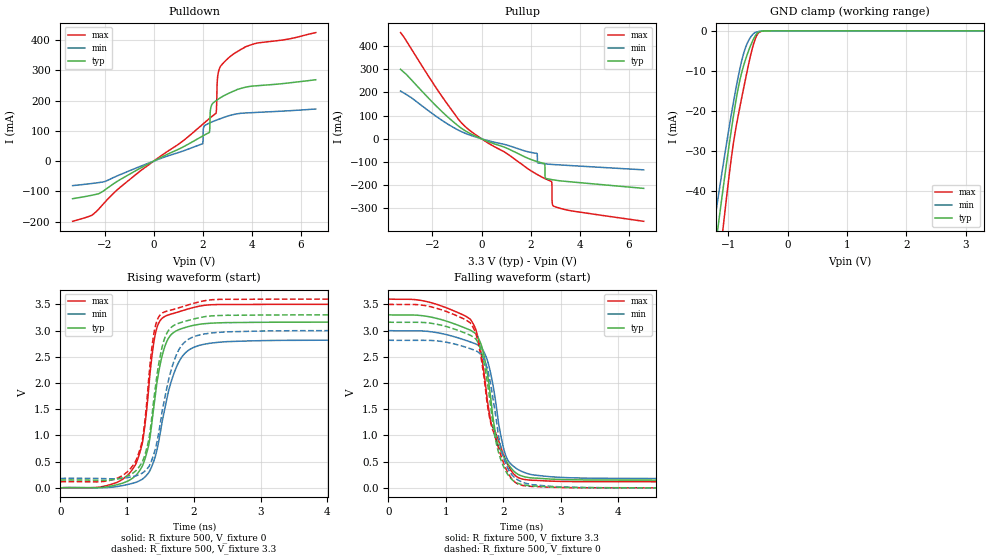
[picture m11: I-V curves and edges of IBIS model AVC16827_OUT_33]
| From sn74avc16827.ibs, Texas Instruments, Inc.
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[Model]   AVC16827_OUT_33
Model_type  3-state
Enable   Active-Low
Vref =   0
Rref =   500
Cref =   30p
Vmeas =   1.5
| variable   typ   min   max
C_comp   4.23pF   3.29pF   5.28pF
| C_pullup   8.79pF   0.04pF   35.28pF
| C_pulldown   16.25pF   1.42pF   50.74pF
| C_tri-state   4.23pF   3.29pF   5.28pF
[Temperature Range]   40   100   -40
| Ambient temperature   25   85   -40
[Voltage range]   3.3   3   3.6
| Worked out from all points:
|   slope of the pulldown table from 0 to 0.495 V, typ, clamps not added: 24.5 ohm
|   slope of the pullup table from 0 to 0.495 V, typ, clamps not added: 23.7 ohm
|   GND clamp passes 1 mA (typ) near -0.53 V on its own axis
|   rising waveform, R_fixture 500, V_fixture 0: 20-80 % time 241ps typ, 309ps min, 207ps max; typ from 0 V to 3.16 V
|   falling waveform, R_fixture 500, V_fixture 3.3: 20-80 % time 293ps typ, 286ps min, 395ps max; typ from 3.3 V to 0.147 V
|   rising waveform, R_fixture 500, V_fixture 3.3: 20-80 % time 223ps typ, 284ps min, 187ps max; typ from 0.147 V to 3.3 V
|   falling waveform, R_fixture 500, V_fixture 0: 20-80 % time 293ps typ, 284ps min, 378ps max; typ from 3.16 V to 0 V
[GND Clamp]
| AVC16827_OUT_33
|   Voltage   I(typ)   I(min)   I(max)
-3.3V     -317.1mA   -273.5mA   -385.8mA
-1.24V    -57.06mA   -48.75mA   -70.66mA
-1.16V    -47.86mA   -40.83mA   -59.48mA
-1.09V    -39.99mA   -34.06mA   -49.94mA
-1.065V   -37.24mA   -31.68mA   -46.61mA
-920mV    -22.15mA   -18.59mA   -28.97mA
-815mV    -13.17mA   -10.31mA   -19.97mA
-695mV    -6.608mA   -3.691mA   -11.11mA
-545mV    -1.293mA   -422.4uA   -2.091mA
-485mV    -308.8uA   -165.9uA   -442.3uA
-370mV    -14.24uA   -20.34uA   -8.566uA
3.3V      1.011nA    10.75nA    48.47pA
[Pulldown]
| AVC16827_OUT_33
|   Voltage   I(typ)   I(min)   I(max)
-3.3V     -124.2mA   -80.91mA   -198.9mA
-2.49V    -112.4mA   -73.57mA   -177.6mA
1.99V     82.86mA    57.31mA    121.5mA
2.04V     85.11mA    112.8mA    125mA
2.265V    94.6mA     125.8mA    140.6mA
2.325V    175.9mA    128.1mA    144.7mA
2.53V     199.3mA    135mA      157.7mA
2.555V    200.8mA    135.7mA    168.3mA
2.59V     202.8mA    136.7mA    264.1mA
2.65V     206.1mA    138.5mA    298.9mA
3.165V    228.4mA    152.5mA    349.4mA
6.6V      269.3mA    172.6mA    425.4mA
[Pullup]
| AVC16827_OUT_33
|   Voltage   I(typ)   I(min)   I(max)
-3.3V     300mA      206.1mA    458.6mA
-735mV    39.21mA    26.92mA    59.95mA
2.255V    -98.1mA    -63.13mA   -153.5mA
2.28V     -98.9mA    -103mA     -155mA
2.565V    -106.8mA   -107.8mA   -170.9mA
2.595V    -168.1mA   -108.1mA   -172.4mA
2.85V     -176mA     -110.5mA   -184.7mA
2.865V    -176.3mA   -110.6mA   -197.1mA
2.87V     -176.4mA   -110.7mA   -265.4mA
2.875V    -176.5mA   -110.7mA   -275.7mA
2.925V    -177.3mA   -111.1mA   -290.3mA
6.6V      -213.9mA   -134mA     -356.1mA
[Ramp]
| AVC16827_OUT_33
| variable   typ   min   max
dV/dt_r   1.90/2.48E-10   1.69/3.13E-10   2.10/2.13E-10
dV/dt_f   1.89/3.01E-10   1.69/2.87E-10   2.09/4.01E-10
R_load = 500
[Rising Waveform]
| AVC16827_OUT_33
R_fixture =   500
C_fixture =   0
L_fixture =   0
V_fixture =   0
V_fixture_min = 0
V_fixture_max = 0
|   Time   V(typ)   V(min)   V(max)
0s        28.92nV    102.8nV    1.632nV
945ps     95.72mV    46.96mV    176.1mV
1.14ns    250mV      109.9mV    486.6mV
1.265ns   544.8mV    206.1mV    1.181V
1.385ns   1.395V     460.4mV    2.642V
1.475ns   2.221V     898mV      3.148V
1.6ns     2.808V     1.724V     3.29V
1.775ns   3.018V     2.402V     3.359V
2.245ns   3.14V      2.759V     3.492V
50ns      3.161V     2.817V     3.501V
[Falling Waveform]
| AVC16827_OUT_33
R_fixture =   500
C_fixture =   0
L_fixture =   0
V_fixture =   3.3
V_fixture_min = 3
V_fixture_max = 3.6
|   Time   V(typ)   V(min)   V(max)
0s        3.3V       3V         3.6V
1.425ns   3.008V     2.783V     3.216V
1.53ns    2.926V     2.74V      2.984V
1.63ns    2.671V     2.655V     2.447V
1.8ns     1.52V      2.07V      1.189V
1.895ns   870.4mV    1.407V     964.3mV
2.055ns   500.6mV    577.2mV    491.5mV
2.23ns    274.8mV    366.8mV    215.2mV
2.5ns     188mV      249.9mV    144.2mV
50ns      146.9mV    177.3mV    115.9mV
[Rising Waveform]
| AVC16827_OUT_33
R_fixture =   500
C_fixture =   0
L_fixture =   0
V_fixture =   3.3
V_fixture_min = 3
V_fixture_max = 3.6
|   Time   V(typ)   V(min)   V(max)
0s        146.9mV    177.3mV    115.9mV
965ps     205.8mV    187.7mV    266.4mV
1.16ns    368.3mV    242.2mV    612.3mV
1.27ns    648.8mV    326.1mV    1.329V
1.38ns    1.471V     566.2mV    2.765V
1.47ns    2.338V     1.03V      3.252V
1.585ns   2.924V     1.846V     3.367V
1.775ns   3.141V     2.634V     3.434V
2.325ns   3.285V     2.961V     3.593V
50ns      3.3V       3V         3.6V
[Falling Waveform]
| AVC16827_OUT_33
R_fixture =   500
C_fixture =   0
L_fixture =   0
V_fixture =   0
V_fixture_min = 0
V_fixture_max = 0
|   Time   V(typ)   V(min)   V(max)
0s        3.161V     2.817V     3.501V
740ps     3.14V      2.812V     3.454V
1.425ns   2.911V     2.654V     3.145V
1.57ns    2.74V      2.582V     2.725V
1.715ns   2.054V     2.295V     1.629V
1.85ns    989.7mV    1.49V      986.3mV
2.005ns   399.8mV    577.9mV    469.1mV
2.2ns     114.4mV    190.6mV    110.1mV
2.5ns     35.19mV    60.29mV    26.11mV
50ns      26.96nV    120.4nV    906.5pV
